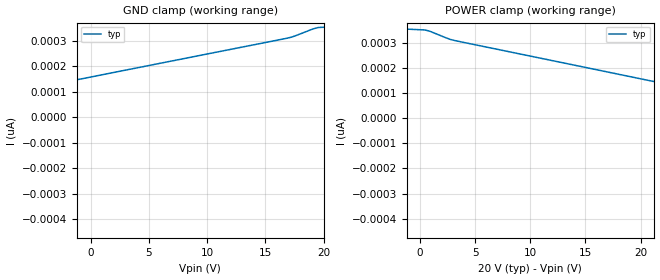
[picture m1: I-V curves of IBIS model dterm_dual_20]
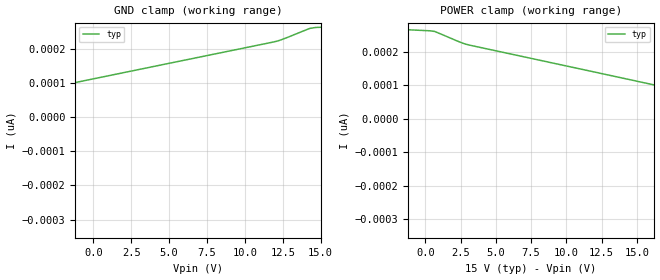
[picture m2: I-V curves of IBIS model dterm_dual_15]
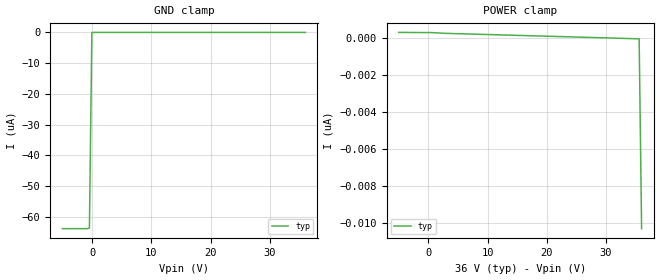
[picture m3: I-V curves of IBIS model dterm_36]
|Texas Instruments Incorporated
|tmux7436f, 2 Data Lane 2:1 44V Precision mux
[IBIS Ver]   4.1
[File name]   tmux7436f.ibs
[Date]   08/04/22
[File Rev]   1.0
[Source]
| Texas Instruments Incorporated.
| ASC-INT-MPD
| 12500 TI Blvd
| Dallas, TX - 75243
[Notes]   Revision History:
| Rev 1.0: 08/04/22
| - Initial version of the model
| - Model generated from simulations in SPECTRE
| - C_comp although listed in numerical order of value are
|   obtained from varying PVT conditions. For PVT conditions for
|   each specific value refer the buffer description under
|   respective [Model]. IBIS model user is responsible for using
|   appropriate C_comp to simulate for Signal Integrity.
[Disclaimer]
| This model is designed as an aid for customers of Texas Instruments.
| TI and its licensors and suppliers make no warranties, either expressed
| or implied, with respect to this  model, including the warranties of
| merchantability or fitness for a particular purpose. The model is
| provided solely on an "as is" basis. The entire risk as to its quality
| and performance is with the customer.
| This model is subject to change without notice. Texas Instruments
| Incorporated is not responsible for updating this model.
[Copyright]
(C) Copyright 2022 Texas Instruments Incorporated.All rights reserved.
|  Component TMUX7436FPW 16-pin - PW package
|  Part # TMUX7436FPW
[Component]   TMUX7436FPW
[Manufacturer]  TI
[Package]
|   typ   min   max
R_pkg   0.0668   NA   NA
L_pkg   2.1992nH   NA   NA
C_pkg   0.2884pF   NA   NA
[Pin]   signal_name   model_name
   1   SEL1   inbuf
   2   S1A   sterm
   3   D1   dterm
   4   S1B   sterm
   5   VSS   power
   6   GND   gnd
   7   NC   nc
   8   DR   inbuf
   9   SEL2   inbuf
   10   S2A   sterm
   11   D2   dterm
   12   S2B   sterm
   13   VDD   power
   14   EN   inbuf
   15   FF   outbuf_od
   16   SF   outbuf_od
[Series Switch Groups]
On 1 /
On 2 /
On 3 /
On 4 /
Off 1 /
[Series Pin Mapping]  pin_2 model_name function_table_group
|   4   3   switch_dual_20   1
|  12  11   switch_dual_20   1
|   2   3   switch_dual_20   2
|  12  11   switch_dual_20   2
|   4   3   switch_dual_20   3
|  10  11   switch_dual_20   3
|   2   3   switch_dual_20   4
|  10  11   switch_dual_20   4
|   4   3   switch_dual_15   1
|  12  11   switch_dual_15   1
|   2   3   switch_dual_15   2
|  12  11   switch_dual_15   2
|   4   3   switch_dual_15   3
|  10  11   switch_dual_15   3
|   2   3   switch_dual_15   4
|  10  11   switch_dual_15   4
|   4   3   switch_36   1
|  12  11   switch_36   1
|   2   3   switch_36   2
|  12  11   switch_36   2
|   4   3   switch_36   3
|  10  11   switch_36   3
|   2   3   switch_36   4
|  10  11   switch_36   4
   4   3   switch_12   1
  12  11   switch_12   1
   2   3   switch_12   2
  12  11   switch_12   2
   4   3   switch_12   3
  10  11   switch_12   3
   2   3   switch_12   4
  10  11   switch_12   4
|  Component TMUX7436FRRP 16-pin - RRP package
|  Part # TMUX7436FRRP
[Component]   TMUX7436FRRP
[Manufacturer]  TI
[Package]
|   typ   min   max
R_pkg   0.0668   NA   NA
L_pkg   2.1992nH   NA   NA
C_pkg   0.2884pF   NA   NA
[Pin]   signal_name   model_name
   1   D1   dterm
   2   S1B   sterm
   3   VSS   power
   4   GND   gnd
   5   DR   inbuf
   6   SEL2   inbuf
   7   NC   nc
   8   S2A   sterm
   9   D2   dterm
   10   S2B   sterm
   11   VDD   power
   12   EN   inbuf
   13   FF   outbuf_od
   14   SF   outbuf_od
   15   SEL1   inbuf
   16   S1A   sterm
[Series Switch Groups]
On 1 /
On 2 /
On 3 /
On 4 /
Off 1 /
[Series Pin Mapping]  pin_2 model_name function_table_group
|   2   1   switch_dual_20   1
|  10   9   switch_dual_20   1
|  16   1   switch_dual_20   2
|  10   9   switch_dual_20   2
|   2   1   switch_dual_20   3
|   8   9   switch_dual_20   3
|  16   1   switch_dual_20   4
|   8   9   switch_dual_20   4
|   2   1   switch_dual_15   1
|  10   9   switch_dual_15   1
|  16   1   switch_dual_15   2
|  10   9   switch_dual_15   2
|   2   1   switch_dual_15   3
|   8   9   switch_dual_15   3
|  16   1   switch_dual_15   4
|   8   9   switch_dual_15   4
|   2   1   switch_36   1
|  10   9   switch_36   1
|  16   1   switch_36   2
|  10   9   switch_36   2
|   2   1   switch_36   3
|   8   9   switch_36   3
|  16   1   switch_36   4
|   8   9   switch_36   4
   2   1   switch_12   1
  10   9   switch_12   1
  16   1   switch_12   2
  10   9   switch_12   2
   2   1   switch_12   3
   8   9   switch_12   3
  16   1   switch_12   4
   8   9   switch_12   4
[Model Selector] dterm
dterm_dual_20 Use for operation at +/-20V
dterm_dual_15 Use for operation at +/-15V
dterm_36 Use for operation at 36V
dterm_12 Use for operation at 12V
[Model Selector] outbuf_od
outbuf_od_5 Use for operation at 5V
[Model Selector] sterm
sterm_dual_20 Use for operation at +/-20V
sterm_dual_15 Use for operation at +/-15V
sterm_36 Use for operation at 36V
sterm_12 Use for operation at 12V
[Model Selector] inbuf
inbuf_dual_20 Use for operation at +/-20V
inbuf_dual_15 Use for operation at +/-15V
inbuf_36 Use for operation at 36V
inbuf_12 Use for operation at 12V
| switch_dual_20
[Model]   switch_dual_20
Model_type   Series_switch
|   typ   min   max
C_comp   4.014581e-12   NA   NA
[Voltage Range]   20   NA   NA
[Power Clamp Reference]   20   NA   NA
[Temperature Range]   27   NA   NA
[On]
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[Off]
|   typ   min   max
[R Series]   10G   NA   NA
| switch_dual_15
[Model]   switch_dual_15
Model_type   Series_switch
|   typ   min   max
C_comp   4.014581e-12   NA   NA
[Voltage Range]   15   NA   NA
[Power Clamp Reference]   15   NA   NA
[Temperature Range]   27   NA   NA
[On]
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[Off]
|   typ   min   max
[R Series]   10G   NA   NA
| switch_36
[Model]   switch_36
Model_type   Series_switch
|   typ   min   max
C_comp   4.014581e-12   NA   NA
[Voltage Range]   36   NA   NA
[Power Clamp Reference]   36   NA   NA
[Temperature Range]   27   NA   NA
[On]
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[Off]
|   typ   min   max
[R Series]   10G   NA   NA
| switch_12
[Model]   switch_12
Model_type   Series_switch
|   typ   min   max
C_comp   4.014581e-12   NA   NA
[Voltage Range]   12   NA   NA
[Power Clamp Reference]   12   NA   NA
[Temperature Range]   27   NA   NA
[On]
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[Off]
|   typ   min   max
[R Series]   10G   NA   NA
| Models and submodels in the file (17): dterm_dual_20 (Terminator), dterm_dual_15 (Terminator), dterm_36 (Terminator), dterm_12 (Terminator), outbuf_od_5 (Open_drain), switch_dual_20 (Series_switch), switch_dual_15 (Series_switch), switch_36 (Series_switch), switch_12 (Series_switch), sterm_dual_20 (Terminator), sterm_dual_15 (Terminator), sterm_36 (Terminator), sterm_12 (Terminator), inbuf_dual_20 (Input), inbuf_dual_15 (Input), inbuf_36 (Input), inbuf_12 (Input)
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| dterm_dual_20
[Model]   dterm_dual_20
Model_type   Terminator
|   typ   min   max
C_comp   4.014581e-12   NA   NA
[Voltage Range]   20   NA   NA
[Temperature Range]   27   NA   NA
[Power Clamp Reference]   20   NA   NA
[GND Clamp Reference]   0   NA   NA
[GND Clamp]
|   Voltage   I(typ)   I(min)   I(max)
-25V      -63.89uA   NA         NA
-20V      -10.3nA    NA         NA
-19.55V   -22.3pA    NA         NA
16.82V    309pA      NA         NA
19.09V    345.8pA    NA         NA
20V       352.4pA    NA         NA
[POWER Clamp]
|   Voltage   I(typ)   I(min)   I(max)
-5V       362.5pA    NA         NA
454.5mV   351.5pA    NA         NA
3.182V    309pA      NA         NA
39.55V    -22.3pA    NA         NA
40V       -10.3nA    NA         NA
| dterm_dual_15
[Model]   dterm_dual_15
Model_type   Terminator
|   typ   min   max
C_comp   4.014581e-12   NA   NA
[Voltage Range]   15   NA   NA
[Temperature Range]   27   NA   NA
[Power Clamp Reference]   15   NA   NA
[GND Clamp Reference]   0   NA   NA
[GND Clamp]
|   Voltage   I(typ)   I(min)   I(max)
-20V      -63.89uA   NA         NA
-15.05V   -71.99nA   NA         NA
-14.7V    -23.81pA   NA         NA
11.82V    218.8pA    NA         NA
12.53V    227.9pA    NA         NA
14.29V    259.2pA    NA         NA
15V       262.5pA    NA         NA
[POWER Clamp]
|   Voltage   I(typ)   I(min)   I(max)
-5V       272.6pA    NA         NA
656.6mV   260pA      NA         NA
2.424V    228.7pA    NA         NA
3.131V    219.3pA    NA         NA
29.65V    -23.26pA   NA         NA
30V       -10.3nA    NA         NA
| dterm_36
[Model]   dterm_36
Model_type   Terminator
|   typ   min   max
C_comp   4.014581e-12   NA   NA
[Voltage Range]   36   NA   NA
[Temperature Range]   27   NA   NA
[Power Clamp Reference]   36   NA   NA
[GND Clamp Reference]   0   NA   NA
[GND Clamp]
|   Voltage   I(typ)   I(min)   I(max)
-5V       -63.89uA   NA         NA
-444.4mV  -63.69uA   NA         NA
-30.3mV   -33.06nA   NA         NA
36V       316.5pA    NA         NA
[POWER Clamp]
|   Voltage   I(typ)   I(min)   I(max)
-5V       326.6pA    NA         NA
383.8mV   316.7pA    NA         NA
35.59V    -22.67pA   NA         NA
36V       -10.29nA   NA         NA
